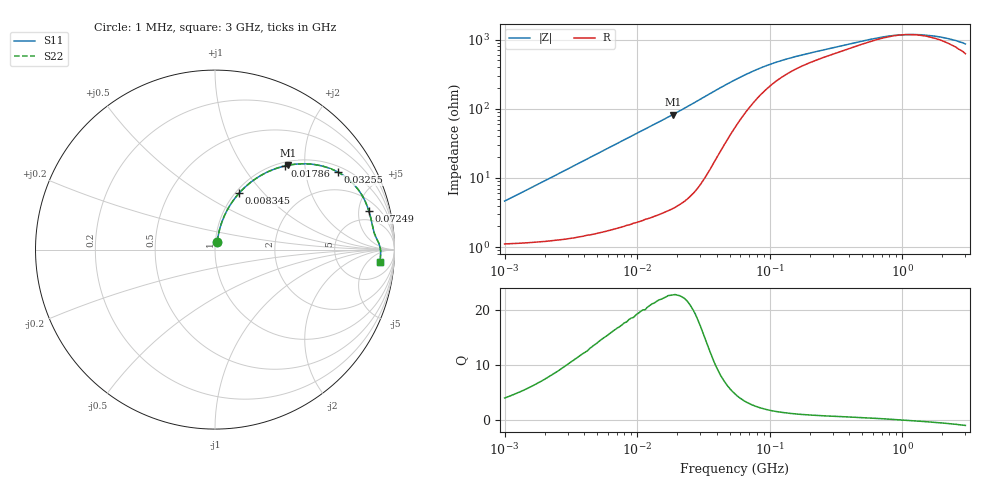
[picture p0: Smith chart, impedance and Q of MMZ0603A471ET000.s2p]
! S-Parameter Data Generated by TDK Corporation
! Copyright(C) 2025 TDK Corporation.
! All Rights Reserved.
! TDK P/N: MMZ0603A471ET000 (Chip Bead)
! Property: |Z|=470ohm at 100MHz
! Size(LxWxT): 0.6x0.3x0.3mm
! Model Type: s2p (Touchstone File Format Version 1.0)
! Frequency: DC=Yes Start=1MHz Stop=3000MHz 202points Log-sweep
! Model Generated on Feb. 6, 2025
! Terms and conditions regarding TDK Simulation Models:
! 1)This simulation model is being provided solely for informational
!  purposes. Please refer to the specifications of the products in
!  terms of detailed characteristics of such products.
! 2)In no event shall TDK Corporation of any of its subsidiaries be
!  liable for any loss or damage arising, directly or indirectly,
!  from any information contained in this simulation model, including,
!  but not limited to loss or damages arising from any inaccuracies,
!  omissions or errors in connection with such information.
! 3)Any and all copyrights on this simulation model are owned by
!  TDK Corporation.  Duplication or redistribution of this simulation
!  model without prior written permission from TDK Corporation
!  is prohibited.
! 4)This simulation model is subject to any modification or change
!  without any prior notice.
! 5)Neither TDK Corporation nor any of its subsidiaries shall make any
!  warranty, express or implied, including but not limited to the
!  correctness, implied warranties of merchantability and fitness for
!  a particular purpose with respect to this simulation models.
! 6)The use of this simulation model shall be deemed to have consented
!  to the terms and conditions hereof.
! Port Assignments:
!  1 ---@@@--- 2
! Applicable Conditions:
!  Temperature = 25 degC
!  DC Bias Current = 0 A
!  Small Signal Operation
# Hz S MA R 50
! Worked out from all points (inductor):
!   201 points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, 1 MHz to 3 GHz, reference 50 ohm
!   read as one part in series: L = 716 nH near 1.041 MHz
!   highest Q = 22.7 at 18.58 MHz (marker M1), where L = 705 nH
!   self-resonance near 1.061 GHz
!   S11 on the Smith chart (normalised r, x): 1 MHz: 1.02, +0.09; 8.345 MHz: 1.04, +0.74; 17.86 MHz: 1.07, +1.58; 32.55 MHz: 1.20, +3.01; 72.49 MHz: 3.24, +6.42; 3 GHz: 14, -12
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1000000  0.04582 73.6  0.988 -2.5  0.988 -2.5  0.04582 73.6
2055611  0.0916 77.3  0.9839 -5.2  0.9839 -5.2  0.0916 77.3
3900413  0.1699 75.5  0.9716 -9.7  0.9716 -9.7  0.1699 75.5
5820586  0.2471 72.0  0.953 -14.3  0.953 -14.3  0.2471 72.0
8345207  0.3407 66.9  0.9213 -19.9  0.9213 -19.9  0.3407 66.9
1.104425e7  0.4301 61.7  0.8816 -25.4  0.8816 -25.4  0.4301 61.7
1.461624e7  0.5313 55.3  0.8232 -32.1  0.8232 -32.1  0.5313 55.3
1.785516e7  0.6074 50.1  0.7681 -37.4  0.7681 -37.4  0.6074 50.1
1.858443e7  0.6227 49.0  0.7556 -38.5  0.7556 -38.5  0.6227 49.0
2.459509e7  0.7252 40.9  0.6553 -46.4  0.6553 -46.4  0.7252 40.9
3.254976e7  0.8084 32.4  0.5367 -53.8  0.5367 -53.8  0.8084 32.4
4.138676e7  0.8524 25.6  0.4349 -57.9  0.4349 -57.9  0.8524 25.6
5.477226e7  0.8764 19.1  0.3345 -59.1  0.3345 -59.1  0.8764 19.1
7.248696e7  0.8838 14.2  0.2598 -56.6  0.2598 -56.6  0.8838 14.2
1.171891e8  0.8871 8.8  0.1831 -47.7  0.1831 -47.7  0.8871 8.8
2.136344e8  0.8949 5.3  0.1363 -36.9  0.1363 -36.9  0.8949 5.3
5.583748e8  0.9146 2.0  0.09168 -20.4  0.09168 -20.4  0.9146 2.0
8.005644e8  0.9198 0.9  0.08154 -9.9  0.08154 -9.9  0.9198 0.9
1.194682e9  0.9225 -0.4  0.07773 4.6  0.07773 4.6  0.9225 -0.4
1.581072e9  0.923 -1.3  0.0801 15.4  0.0801 15.4  0.923 -1.3
2.177892e9  0.9228 -2.6  0.0883 27.7  0.0883 27.7  0.9228 -2.6
3e9  0.9202 -4.2  0.1064 39.4  0.1064 39.4  0.9202 -4.2
